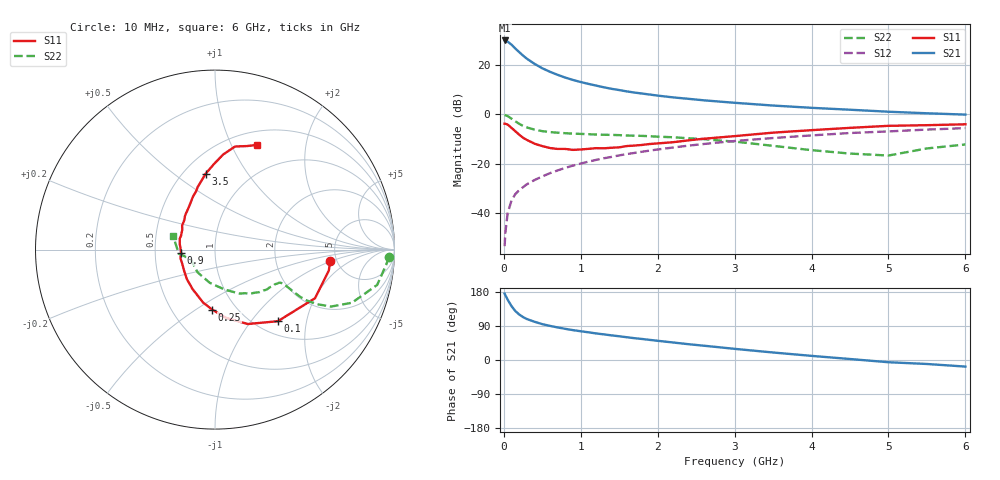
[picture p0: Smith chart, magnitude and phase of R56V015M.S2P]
! SIEMENS Small Signal Semiconductors
! BFR183
! Si NPN RF Bipolar Junction Transistor in SOT23
! VCE = 6 V  IC = 15 mA
! Common Emitter S-Parameters:  May  1996
# GHz  S  MA  R  50
!  f  S11  S21  S12  S22
! GHz  MAG  ANG  MAG  ANG  MAG  ANG  MAG  ANG
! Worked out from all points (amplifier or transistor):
!   36 points, 10 MHz to 6 GHz, reference 50 ohm
!   highest |S21| = 30.0 dB at 10 MHz (marker M1)
!   |S21| within 3 dB of that: start of sweep to 140.5 MHz
!   unconditionally stable (mu >= 1): 680.2 MHz to 2.468 GHz
!   at 250 MHz: K = 0.73, MSG = 26.7 dB, |S12| = -29.6 dB
!   at 1.4 GHz: K = 1.05, MAG = 12.5 dB, |S12| = -17.3 dB
!   at 6 GHz: K = 0.89, MSG = 2.7 dB, |S12| = -5.6 dB
!   S11 on the Smith chart (normalised r, x): 10 MHz: 4.45, -0.93; 100 MHz: 1.24, -1.37; 250 MHz: 0.78, -0.59; 900 MHz: 0.68, -0.02; 3.5 GHz: 0.64, +0.66; 6 GHz: 0.65, +1.26
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0.01  0.6461 -5.4  31.76 175.2  0.0021 90.1  0.9708 -2.4
0.02  0.6446 -10.5  31.24 170.9  0.004 75.7  0.9572 -5.1
0.05  0.6197 -25.9  30.03 159.1  0.0099 79.2  0.9247 -12.3
0.1  0.5309 -48.7  26.08 142.1  0.0179 71.9  0.8186 -21.2
0.15  0.4532 -66.2  21.72 129.1  0.0241 66.2  0.7212 -26.1
0.2  0.3863 -80.6  18.39 120.1  0.0288 66.6  0.6432 -28.2
0.25  0.3349 -92.6  15.63 113.2  0.0332 65.4  0.5827 -29.0
0.3  0.3024 -102.6  13.51 108.1  0.0381 66.2  0.5426 -29.0
0.4  0.2535 -119.4  10.62 100.8  0.0464 67.1  0.4896 -28.1
0.5  0.2267 -133.9  8.642 94.6  0.0548 68.3  0.4562 -27.3
0.6  0.2071 -146.8  7.326 90.0  0.0639 68.7  0.4367 -26.8
0.7  0.1985 -157.5  6.353 85.9  0.0727 69.1  0.4246 -26.7
0.9  0.19 -175.0  5 78.8  0.0912 68.7  0.406 -27.0
1.1  0.1993 170.7  4.164 73.1  0.1096 67.9  0.395 -28.7
1.3  0.2043 157.8  3.55 67.6  0.1281 66.7  0.3852 -30.3
1.6  0.2276 143.6  2.927 60.0  0.1564 64.1  0.3719 -34.2
2.2  0.272 123.5  2.214 46.2  0.2123 58.4  0.3429 -43.7
3.5  0.4255 97.1  1.511 19.8  0.3307 42.9  0.2294 -76.3
4.5  0.5324 85.0  1.243 2.6  0.4182 30.6  0.1598 -127.4
5  0.5851 79.0  1.132 -5.9  0.4508 23.2  0.1458 -158.7
5.5  0.6032 73.0  1.053 -10.5  0.491 19.1  0.2033 -173.8
6  0.6287 68.0  0.989 -17.4  0.5261 11.5  0.2447 162.1
